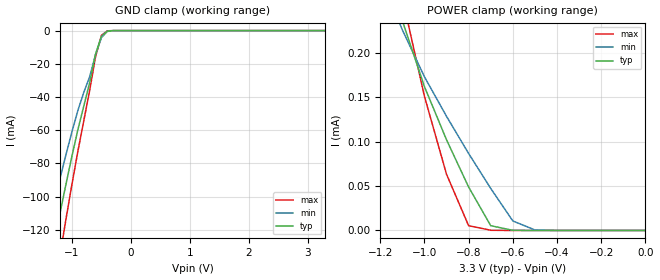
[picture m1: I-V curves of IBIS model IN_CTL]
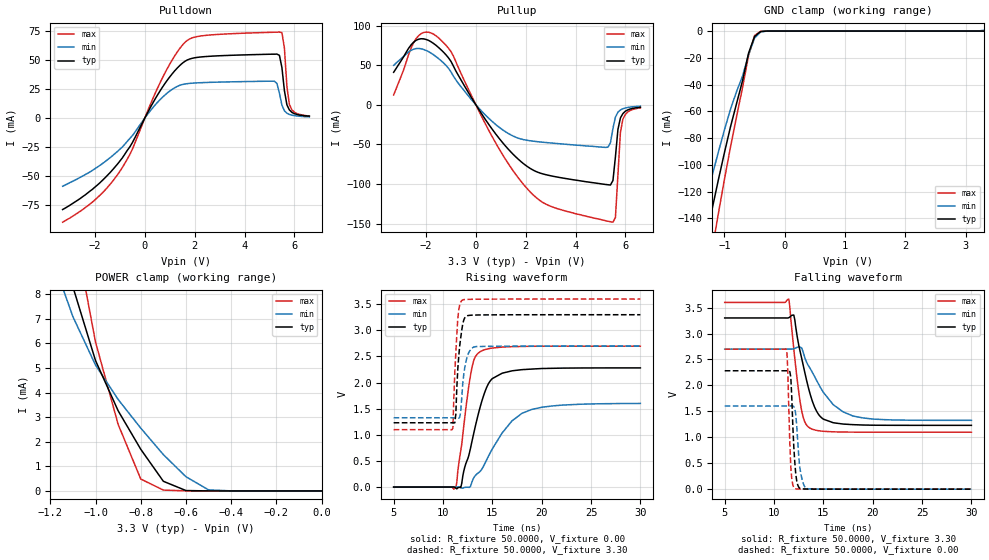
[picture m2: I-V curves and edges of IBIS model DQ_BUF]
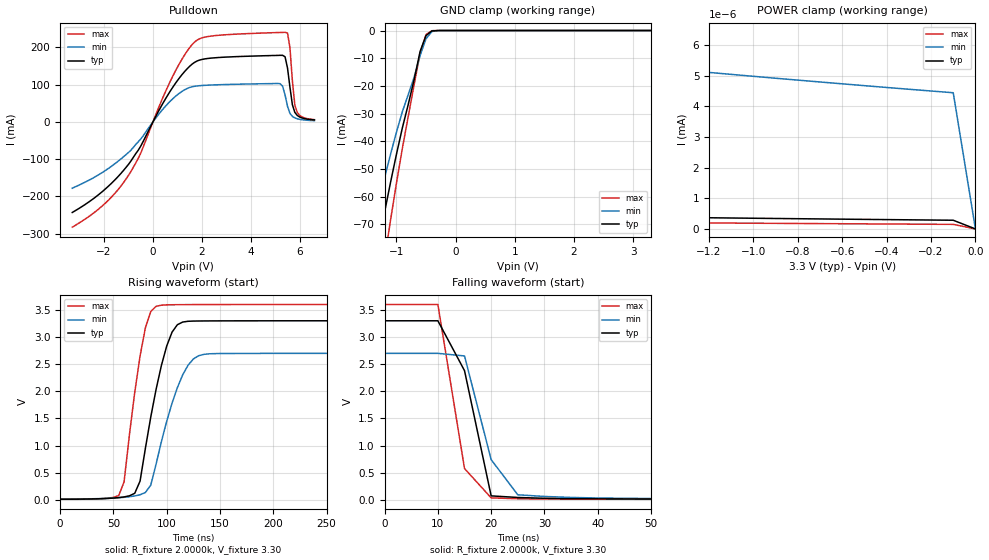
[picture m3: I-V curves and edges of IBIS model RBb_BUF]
| This IBIS file was created by s2ibis3 version 1.1
| North Carolina State University, ERL, 2006
[IBIS ver] 3.2
[File name] s34ml02g2_b_i_33_r3.ibs
[File Rev] 3.0
|   Rev1.0 Initial release (X16 ONFI F32 98799AB 41087)
|   Rev2.0 Update with measurement
|   Rev3.0 Update 0A for 0V
[Date] 7/23/2014
[Source] Spansion IBIS team
|   Email: dl.ibisteam@spansion.com
[Notes]  Generated IBIS models from SPICE simulations.
|   VIO=3.3V, Temperature Range: Industrial (-40oC to +90oC).
[Disclaimer] THE MODEL LIBRARIES ARE PROVIDED AS IS.
[Copyright] (C) COPYRIGHT 2014
| SPANSION LLC
| ALL RIGHTS RESERVED.
|   Component S34ML02G2 X16 ONFI F32 in VBM063 package
[Component]   S34ML02G2
[Manufacturer]   Spansion
[Package]
| variable   typ   min   max
R_pkg   302.04mOhm   265.58mOhm   343.49mOhm
L_pkg   6.92nH   5.79nH   8.79nH
C_pkg   0.76pF   0.55pF   0.86pF
[Pin]   signal_name   model_name   R_pin   L_pin   C_pin
A1   R   NC
A2   R   NC
A9   R   NC
A10   R   NC
B1   R   NC
B9   R   NC
B10   R   NC
C3   WP#   IN_CTL   343.49m   8.79n   0.80p
C4   ALE   IN_CTL   330.54m   7.73n   0.86p
C5   VSS   GND
C6   CE#   IN_CTL   294.66m   6.65n   0.74p
C7   WE#   IN_CTL   315.12m   7.33n   0.85p
C8   RB#   RBb_BUF   270.20m   6.56n   0.70p
D3   VDD   POWER
D4   RE#   IN_CTL   336.66m   8.33n   0.74p
D5   CLE   IN_CTL   278.71m   6.08n   0.78p
D6   R   NC
D7   R   NC
D8   R   NC
E3   R   NC
E4   R   NC
E5   R   NC
E6   R   NC
E7   R   NC
E8   R   NC
F3   R   NC
F4   R   NC
F5   R   NC
F6   R   NC
F7   VSS   GND
F8   R   NC
G3   R   NC
G4   VDD   POWER
G5   R   NC
G6   I/O13   DQ_BUF   292.34m   7.15n   0.76p
G7   I/O15   DQ_BUF   292.72m   6.22n   0.79p
G8   R   NC
H3   I/O8   DQ_BUF   318.53m   6.98n   0.82p
H4   I/O0   DQ_BUF   316.27m   6.62n   0.80p
H5   I/O10   DQ_BUF   265.58m   5.79n   0.55p
H6   I/O12   DQ_BUF   303.2m   7.22n   0.84p
H7   I/O14   DQ_BUF   282.94m   6.57n   0.77p
H8   VDD   POWER
J3   I/O9   DQ_BUF   322.17m   7.36n   0.80p
J4   I/O1   DQ_BUF   299.18m   6.36n   0.62p
J5   I/O11   DQ_BUF   288.33m   6.83n   0.68p
J6   VDD   POWER
J7   I/O5   DQ_BUF   282.95m   6.78n   0.67p
J8   I/O7   DQ_BUF   297.23m   6.80n   0.71p
K3   VSS   GND
K4   I/O2   DQ_BUF   327.47m   7.16n   0.86p
K5   I/O3   DQ_BUF   279.82m   6.26n   0.72p
K6   I/O4   DQ_BUF   307.00m   6.80n   0.83p
K7   I/O6   DQ_BUF   301.73m   6.91n   0.75p
K8   VSS   GND
L1   R   NC
L2   R   NC
L9   R   NC
L10   R   NC
M1   R   NC
M2   R   NC
M9   R   NC
M10   R   NC
| Models and submodels in the file (3): IN_CTL (Input), DQ_BUF (I/O), RBb_BUF (Open_drain)
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|   Model IN_CTL
[Model]   IN_CTL
Model_type   Input
Vinl =   1.3180
Vinh =   1.6630
C_comp   6.01pF   5.78pF   8.57pF
[Temperature Range]   25.0000   90.0000   -40.0000
[Voltage Range]   3.3000   2.7000   3.6000
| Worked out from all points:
|   GND clamp passes 1 mA (typ) near -0.42 V on its own axis
|   POWER clamp passes 1 mA (typ) near -1.80 V on its own axis
[GND_clamp]
| voltage   I(typ)   I(min)   I(max)
-3.3V     -563.9mA   -475.7mA   -665.6mA
-1.5V     -164.8mA   -133.7mA   -202.4mA
-1.4V     -145.8mA   -118.2mA   -179.3mA
-1.3V     -127.4mA   -103.2mA   -156.7mA
-1.2V     -109.5mA   -88.65mA   -134.7mA
-1.1V     -92.25mA   -74.51mA   -113.2mA
-900mV    -59.75mA   -48.15mA   -72.81mA
-700mV    -31.42mA   -27.84mA   -36.18mA
-600mV    -14.17mA   -14.52mA   -15.79mA
-500mV    -3.458mA   -4.259mA   -2.945mA
-400mV    -298.7uA   -518.7uA   -127.7uA
3.3V      292.5pA    10.73uA    139.6pA
[POWER_clamp]
| voltage   I(typ)   I(min)   I(max)
-3.3V     27.06A     13.23A     34.66A
-1.1V     236.4uA    226.1uA    262.5uA
-1V       162.2uA    173.2uA    151.3uA
-900mV    102.2uA    128.6uA    63.39uA
-800mV    48.96uA    86.76uA    5.425uA
-700mV    5.388uA    47.41uA    237.2nA
-600mV    176.5nA    10.73uA    6.564nA
-500mV    6.019nA    596nA      279.6pA
0V        0A         0A         0A
|   Model DQ_BUF
[Model]   DQ_BUF
Model_type   I/O
Polarity   Non-Inverting
Enable   Active-High
Vinl =   1.3180
Vinh =   1.6630
Vmeas =   1.65V
C_comp   2.54pF   2.48pF   2.73pF
[Temperature Range]   25.0000   90.0000   -40.0000
[Voltage Range]   3.3000   2.7000   3.6000
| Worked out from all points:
|   slope of the pulldown table from 0 to 0.495 V, typ, clamps not added: 25.6 ohm
|   slope of the pullup table from 0 to 0.495 V, typ, clamps not added: 20.9 ohm
|   GND clamp passes 1 mA (typ) near -0.42 V on its own axis
|   POWER clamp passes 1 mA (typ) near -0.75 V on its own axis
|   rising waveform, R_fixture 50.0000, V_fixture 0.00: 20-80 % time 1.92ns typ, 3.23ns min, 1.14ns max; typ from 0 V to 2.28 V
|   rising waveform, R_fixture 50.0000, V_fixture 3.30: 20-80 % time 465ps typ, 496ps min, 379ps max; typ from 1.23 V to 3.3 V
|   falling waveform, R_fixture 50.0000, V_fixture 3.30: 20-80 % time 1.58ns typ, 2.84ns min, 926ps max; typ from 3.3 V to 1.23 V
|   falling waveform, R_fixture 50.0000, V_fixture 0.00: 20-80 % time 346ps typ, 421ps min, 262ps max; typ from 2.28 V to 0 V
[GND_clamp]
| voltage   I(typ)   I(min)   I(max)
-3.3V     -1.531A    -857.2mA   -2.572A
-1.5V     -199.4mA   -161.9mA   -246.1mA
-1.4V     -176.3mA   -143.2mA   -217.6mA
-1.3V     -153.9mA   -125mA     -189.7mA
-1.2V     -132.2mA   -107.4mA   -162.6mA
-1.1V     -111.1mA   -90.32mA   -136.3mA
-900mV    -71.7mA    -58.5mA    -86.72mA
-700mV    -37.18mA   -33.68mA   -42.32mA
-600mV    -16.53mA   -17.62mA   -18.35mA
-500mV    -4.024mA   -5.179mA   -3.39mA
-400mV    -347uA     -622.1uA   -145.7uA
3.3V      401pA      577.4uA    196.4pA
[POWER_clamp]
| voltage   I(typ)   I(min)   I(max)
-3.3V     28.02A     13.67A     36.43A
-1.2V     12.2mA     9.687mA    16.8mA
-1.1V     8.304mA    7.091mA    10.97mA
-1V       5.304mA    5.122mA    6.06mA
-900mV    3.262mA    3.722mA    2.71mA
-800mV    1.696mA    2.556mA    484.6uA
-700mV    392.2uA    1.477mA    34.23uA
-600mV    15.16uA    577.4uA    1.674uA
-500mV    621.3nA    42.06uA    41.77nA
-400mV    23.44nA    2.247uA    920.4pA
0V        0A         0A         0A
[Pulldown]
| voltage   I(typ)   I(min)   I(max)
-3.3V     -78.9mA    -58.8mA    -89.8mA
-1.1V     -39.8mA    -28.88mA   -49mA
-500mV    -21.23mA   -15.18mA   -26.87mA
900mV     32.53mA    21.5mA     42.55mA
1.8V      50.8mA     29.79mA    68.12mA
5.2V      54.94mA    31.61mA    73.89mA
5.4V      53.96mA    21.3mA     73.98mA
5.5V      43.4mA     11.1mA     73.57mA
5.6V      23.6mA     6.2mA      60.2mA
5.7V      11.3mA     4.1mA      27.2mA
5.8V      6.9mA      3mA        11.6mA
6.6V      1.6mA      900uA      1.8mA
[Pullup]
| voltage   I(typ)   I(min)   I(max)
-3.3V     41mA       49.8mA     12.4mA
-2.4V     81.3mA     70.88mA    83.4mA
-1.7V     77.37mA    63.08mA    89.09mA
-1V       54.74mA    41.53mA    67.09mA
700mV     -32.73mA   -22.28mA   -42.8mA
2.2V      -80.59mA   -45.42mA   -110.5mA
5.3V      -100.8mA   -53.4mA    -146.8mA
5.5V      -95.4mA    -29.8mA    -148mA
5.6V      -65.2mA    -15.4mA    -141.9mA
5.8V      -16.5mA    -6.5mA     -34.4mA
5.9V      -11mA      -4.9mA     -18mA
6.6V      -3.1mA     -1.7mA     -3.9mA
[Ramp]
| variable   typ   min   max
dV/dt_r   2.2818/1.922e-09   1.6009/3.212e-09   2.6978/1.138e-09
dV/dt_f   2.0696/1.584e-09   1.3732/2.799e-09   2.5018/9.242e-10
R_load = 50.0000
[Rising Waveform]
R_fixture = 50.0000
V_fixture = 0.00
| time   V(typ)   V(min)   V(max)
5ns       0V         0V         0V
11.3ns    -21.43mV   33.17uV    -13.34mV
11.8ns    -8.737mV   -10.81mV   695.5mV
12.9ns    842.8mV    76.14mV    2.255V
13.3ns    1.182V     224.4mV    2.504V
13.9ns    1.621V     332.1mV    2.606V
15ns      2.077V     731mV      2.662V
18ns      2.248V     1.411V     2.692V
22ns      2.277V     1.568V     2.697V
30ns      2.282V     1.601V     2.698V
[Rising Waveform]
R_fixture = 50.0000
V_fixture = 3.30
V_fixture_min = 2.70
V_fixture_max = 3.60
| time   V(typ)   V(min)   V(max)
5ns       1.23V      1.327V     1.098V
11ns      1.23V      1.327V     1.126V
11.2ns    1.231V     1.327V     2.214V
11.3ns    1.394V     1.327V     2.572V
11.5ns    2.262V     1.322V     3.228V
11.8ns    2.866V     1.452V     3.546V
12ns      3.122V     1.977V     3.582V
12.5ns    3.283V     2.523V     3.594V
13.2ns    3.294V     2.685V     3.596V
30ns      3.3V       2.7V       3.6V
[Falling Waveform]
R_fixture = 50.0000
V_fixture = 3.30
V_fixture_min = 2.70
V_fixture_max = 3.60
| time   V(typ)   V(min)   V(max)
5ns       3.3V       2.7V       3.6V
11.5ns    3.305V     2.7V       3.664V
12ns      3.357V     2.706V     2.703V
12.7ns    2.606V     2.733V     1.617V
13.1ns    2.264V     2.547V     1.304V
13.7ns    1.805V     2.313V     1.171V
14.3ns    1.507V     2.101V     1.134V
15ns      1.35V      1.866V     1.115V
18ns      1.244V     1.41V      1.1V
30ns      1.23V      1.327V     1.098V
[Falling Waveform]
R_fixture = 50.0000
V_fixture = 0.00
| time   V(typ)   V(min)   V(max)
5ns       2.282V     1.603V     2.698V
11.3ns    2.282V     1.603V     2.671V
11.4ns    2.283V     1.603V     2.243V
11.6ns    2.265V     1.603V     880.5mV
11.7ns    2.158V     1.605V     421.3mV
12.1ns    524.6mV    1.55V      10mV
12.3ns    158.3mV    1.219V     4.58mV
12.6ns    17.13mV    438.4mV    2.749mV
13.3ns    2.691mV    14.67mV    1.287mV
30ns      0V         641.2nV    0V
|   Model RBb_BUF
[Model]   RBb_BUF
Model_type   Open_drain
Polarity   Non-Inverting
Enable   Active-High
Vmeas =   1.65V
Rref =  2.0000k
Vref =  3.3000
C_comp   6.45pF   6.07pF   9.98pF
[Temperature Range]   25.0000   90.0000   -40.0000
[Voltage Range]   3.3000   2.7000   3.6000
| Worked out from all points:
|   slope of the pulldown table from 0 to 0.495 V, typ, clamps not added: 8.28 ohm
|   GND clamp passes 1 mA (typ) near -0.45 V on its own axis
|   POWER clamp passes 1 mA (typ) near -2.01 V on its own axis
|   rising waveform, R_fixture 2.0000k, V_fixture 3.30: 20-80 % time 19.6ns typ, 23.4ns min, 14.9ns max; typ from 0.013 V to 3.3 V
|   falling waveform, R_fixture 2.0000k, V_fixture 3.30: 20-80 % time 5.13ns typ, 5.19ns min, 3.56ns max; typ from 3.3 V to 0.013 V
[GND_clamp]
| voltage   I(typ)   I(min)   I(max)
-3.3V     -366.9mA   -293.6mA   -456.9mA
-1.5V     -100.2mA   -80.18mA   -128.1mA
-1.4V     -88.25mA   -70.88mA   -112.4mA
-1.3V     -76.7mA    -61.86mA   -97.26mA
-1.2V     -65.58mA   -53.15mA   -82.61mA
-1.1V     -54.91mA   -44.75mA   -68.56mA
-900mV    -35.17mA   -29.31mA   -42.57mA
-700mV    -17.63mA   -16.78mA   -19.44mA
-600mV    -7.539mA   -8.992mA   -8.14mA
-500mV    -1.807mA   -2.957mA   -1.425mA
-400mV    -154.4uA   -343.9uA   -57.58uA
3.3V      277.7pA    4.735nA    133.2pA
[POWER_clamp]
| voltage   I(typ)   I(min)   I(max)
-3.3V     1.67A      608.7mA    3.4A
-2.1V     9.427mA    14nA       295.6mA
-2V       303.3uA    6.064nA    92.6mA
-1.9V     7.905uA    5.601nA    4.048mA
-1.8V     205nA      5.511nA    40.63uA
-1.7V     5.702nA    5.44nA     380.1nA
-1.6V     535.8pA    5.372nA    3.762nA
-1.5V     393.7pA    5.304nA    242pA
-1.4V     381.8pA    5.237nA    204.8pA
-100mV    284.5pA    4.444nA    149.5pA
0V        0A         0A         0A
[Pulldown]
| voltage   I(typ)   I(min)   I(max)
-3.3V     -243.1mA   -178.1mA   -282.5mA
-1.1V     -122.1mA   -87.85mA   -153.2mA
-500mV    -65.05mA   -46.01mA   -83.83mA
900mV     101.5mA    67.22mA    134.1mA
1.9V      165.6mA    96.88mA    222.7mA
5.2V      178.4mA    102.3mA    239.7mA
5.4V      174.4mA    72.03mA    240.1mA
5.5V      144.4mA    41.6mA     238.5mA
5.6V      92.7mA     22.6mA     198.7mA
5.8V      25.3mA     10.5mA     44.7mA
6V        12.8mA     6.7mA      17.2mA
6.6V      5.1mA      3.2mA      5.9mA
[Ramp]
| variable   typ   min   max
dV/dt_r   2.8332/2.379e-08   2.1685/3.033e-08   3.2023/1.743e-08
dV/dt_f   2.8261/1.790e-08   2.1396/3.173e-08   3.2012/1.043e-08
R_load = 50.0000
[Rising Waveform]
R_fixture = 2.0000k
V_fixture = 3.30
V_fixture_min = 2.70
V_fixture_max = 3.60
| time   V(typ)   V(min)   V(max)
0s        12.68mV    14.86mV    10.59mV
55ns      42.37mV    39.93mV    80.39mV
60ns      55.15mV    47.84mV    332.1mV
75ns      346.4mV    94.68mV    2.651V
80ns      949.9mV    137.4mV    3.171V
90ns      2.033V     656.3mV    3.565V
105ns     3.09V      1.781V     3.595V
120ns     3.291V     2.48V      3.598V
135ns     3.297V     2.682V     3.599V
495ns     3.3V       2.7V       3.6V
[Falling Waveform]
R_fixture = 2.0000k
V_fixture = 3.30
V_fixture_min = 2.70
V_fixture_max = 3.60
| time   V(typ)   V(min)   V(max)
0s        3.3V       2.7V       3.6V
10ns      3.3V       2.7V       3.6V
15ns      2.381V     2.652V     577.9mV
20ns      74.22mV    741.6mV    37.37mV
25ns      44.85mV    94.16mV    21.35mV
30ns      29.93mV    63.6mV     15.81mV
40ns      19.68mV    35.16mV    12.67mV
105ns     13.24mV    16.77mV    10.69mV
495ns     12.68mV    14.86mV    10.59mV
